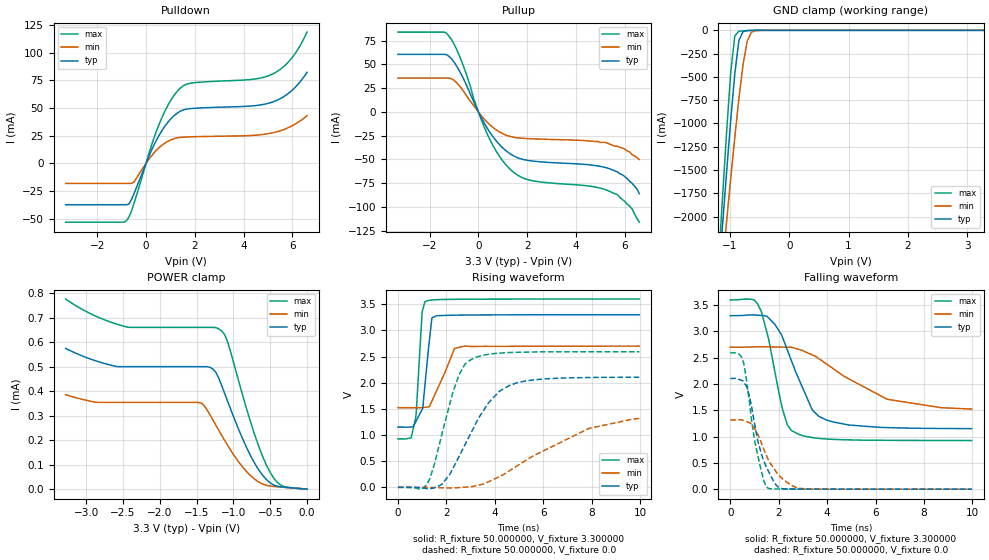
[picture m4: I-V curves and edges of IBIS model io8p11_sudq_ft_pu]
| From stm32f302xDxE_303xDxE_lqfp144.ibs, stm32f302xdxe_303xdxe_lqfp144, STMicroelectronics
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|   Model io8p11_sudq_ft_pu
[Model]  io8p11_sudq_ft_pu
Model_type I/O
Polarity   Non-Inverting
Enable   Active-Low
Vinl =   0.990000V
Vinh =   2.310000V
Vmeas =  1.650000V
Cref =   30.000000pF
Rref =   100.000000M
Vref =   0.0V
C_comp   1.970900pF   1.892300pF   2.063200pF
[Temperature Range]   25.000000   0.125000k   -40.000000
[Pullup Reference]   3.300000V   2.700000V   3.600000V
[Pulldown Reference]   0.0V   0.0V   0.0V
[POWER Clamp Reference]   3.300000V   2.700000V   3.600000V
[GND Clamp Reference]   0.0V   0.0V   0.0V
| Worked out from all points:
|   slope of the pulldown table from 0 to 0.495 V, typ, clamps not added: 20.9 ohm
|   slope of the pullup table from 0 to 0.495 V, typ, clamps not added: 22.2 ohm
|   GND clamp passes 1 mA (typ) near -0.64 V on its own axis
|   rising waveform, R_fixture 50.000000, V_fixture 3.300000: 20-80 % time 276ps typ, 662ps min, 203ps max; typ from 1.15 V to 3.3 V
|   rising waveform, R_fixture 50.000000, V_fixture 0.0: 20-80 % time 1.54ns typ, 3.15ns min, 915ps max; typ from 0.001 V to 2.1 V
|   falling waveform, R_fixture 50.000000, V_fixture 3.300000: 20-80 % time 1.14ns typ, 2.57ns min, 735ps max; typ from 3.3 V to 1.15 V
|   falling waveform, R_fixture 50.000000, V_fixture 0.0: 20-80 % time 662ps typ, 877ps min, 528ps max; typ from 2.1 V to 0.001 V
[Pulldown]
|Voltage   I(typ)   I(min)   I(max)
-3.3V     -37.45mA   -18.2mA    -53.24mA
-800mV    -37.45mA   -18.2mA    -51.9mA
-700mV    -36.7mA    -18.2mA    -48.48mA
-500mV    -27.71mA   -17.01mA   -36.65mA
500mV     23.91mA    13.38mA    33.24mA
900mV     37.17mA    19.88mA    52.48mA
1.3V      45.55mA    23.01mA    65.5mA
1.8V      49.29mA    23.83mA    72.18mA
4.4V      51.88mA    25.21mA    75.91mA
5.2V      55.41mA    27.53mA    80.72mA
5.9V      64.2mA     32.82mA    93.01mA
6.6V      82.13mA    42.97mA    118.5mA
[Pullup]
|Voltage   I(typ)   I(min)   I(max)
-3.3V     60.64mA    35.67mA    84.08mA
-1.4V     60.64mA    35.67mA    84.08mA
-1.2V     58.55mA    35.67mA    79.69mA
-700mV    39.45mA    25.05mA    54.07mA
-100mV    5.36mA     3.465mA    7.201mA
400mV     -18.61mA   -11.78mA   -25.23mA
900mV     -35.28mA   -21.55mA   -48mA
1.5V      -46.91mA   -26.86mA   -64.58mA
2.2V      -51.57mA   -28.22mA   -72.25mA
5.3V      -59.1mA    -33mA      -82.6mA
6.2V      -73mA      -42mA      -99mA
6.6V      -86mA      -50mA      -116mA
[GND_clamp]
|Voltage   I(typ)   I(min)   I(max)
-3.3V     -9.525A    -9.501A    -9.513A
-1.2V     -2.719A    -3.023A    -2.568A
-1.13V    -2.122A    -2.541A    -1.826A
-1.06V    -1.537A    -2.065A    -1.111A
-990mV    -975.7mA   -1.599A    -462mA
-920mV    -467.4mA   -1.149A    -59mA
-850mV    -106.6mA   -727.3mA   -10.11mA
-780mV    -13.06mA   -365.4mA   -5.254mA
-710mV    -3.045mA   -114.8mA   -2.635mA
-640mV    -943.2uA   -20.16mA   -905.7uA
-570mV    -199.4uA   -3.959mA   -156.8uA
3.28V     0A         0A         0A
[POWER_clamp]
|Voltage   I(typ)   I(min)   I(max)
-3.28V    574uA      385.1uA    775.2uA
-2.88V    524.3uA    354.9uA    706.9uA
-2.44V    499.6uA    353.9uA    660.7uA
-1.44V    499.6uA    351.4uA    659.6uA
-1.28V    490.1uA    283.2uA    659.6uA
-1.16V    423.2uA    219.6uA    645uA
-1.08V    359.8uA    179.3uA    602.1uA
-800mV    156.6uA    65uA       306.5uA
-640mV    71.59uA    26.48uA    162uA
-520mV    30.4uA     13.8uA     79.2uA
-360mV    9.635uA    8.674uA    17.24uA
0V        0A         0A         0A
[Ramp]
| variable   typ   min   max
dV/dt_r  1.26186/1.54154n   0.74296/3.12788n   1.55433/0.91415n
dV/dt_f  1.28736/1.14139n   0.68730/2.59063n   1.60397/0.73478n
R_load = 50.000000
[Rising Waveform]
R_fixture= 50.000000
V_fixture= 3.300000
V_fixture_min= 2.700000
V_fixture_max= 3.600000
|time   V(typ)   V(min)   V(max)
0s        1.152V     1.524V     926.8mV
540.5ps   1.154V     1.523V     947.7mV
740.7ps   1.259V     1.522V     1.347V
1.001ns   1.488V     1.526V     3.36V
1.121ns   1.981V     1.531V     3.552V
1.401ns   3.237V     1.647V     3.581V
1.582ns   3.278V     1.831V     3.587V
2.342ns   3.291V     2.658V     3.595V
2.763ns   3.294V     2.702V     3.597V
9.97ns    3.3V       2.7V       3.6V
[Rising Waveform]
R_fixture= 50.000000
V_fixture= 0.0
V_fixture_min= 0.0
V_fixture_max= 0.0
|time   V(typ)   V(min)   V(max)
0s        1.091mV    1.201mV    1.047mV
1.181ns   -22.27mV   208.2uV    48.55mV
1.481ns   -10.34mV   -2.93mV    401.7mV
1.822ns   60.95mV    -7.891mV   1.028V
2.503ns   571.6mV    -4.301mV   2.126V
3.043ns   1.064V     14.13mV    2.448V
3.744ns   1.617V     108.7mV    2.543V
4.905ns   1.998V     405.7mV    2.581V
7.888ns   2.1V       1.127V     2.592V
9.97ns    2.105V     1.317V     2.592V
[Falling Waveform]
R_fixture= 50.000000
V_fixture= 3.300000
V_fixture_min= 2.700000
V_fixture_max= 3.600000
|time   V(typ)   V(min)   V(max)
0s        3.3V       2.7V       3.6V
981ps     3.314V     2.706V     3.602V
1.281ns   3.304V     2.71V      3.38V
1.582ns   3.258V     2.707V     2.86V
2.142ns   2.908V     2.701V     1.552V
2.523ns   2.448V     2.699V     1.118V
3.383ns   1.51V      2.554V     982.3mV
3.984ns   1.314V     2.378V     954.8mV
6.486ns   1.172V     1.709V     929.7mV
9.97ns    1.152V     1.524V     926.8mV
[Falling Waveform]
R_fixture= 50.000000
V_fixture= 0.0
V_fixture_min= 0.0
V_fixture_max= 0.0
|time   V(typ)   V(min)   V(max)
0s        2.105V     1.317V     2.592V
340.3ps   2.093V     1.321V     2.573V
560.6ps   2.035V     1.305V     2.384V
760.8ps   1.822V     1.27V      1.763V
1.021ns   1.205V     1.142V     888.8mV
1.401ns   520.4mV    739.5mV    140.2mV
1.582ns   338mV      548.5mV    15.88mV
2.002ns   34.75mV    265.7mV    3.667mV
2.863ns   3.105mV    18.83mV    2.018mV
9.97ns    1.091mV    1.201mV    1.047mV
